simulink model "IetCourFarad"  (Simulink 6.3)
settings: Solver=ode45  StartTime=0.0  StopTime=5E-4  RelTol=1e-3
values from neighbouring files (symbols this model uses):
  beta = 0.95    [Constantes.m]    (also in ConstantesBck.m; ResCourV1.m = 1; ResCrV1.m = 1; ResEnerV1.m = 1)
undefined symbols (not defined in the file or in its folder): ln
libraries: simulink x1

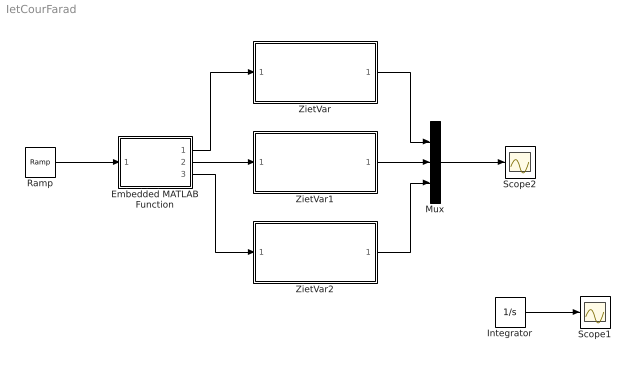
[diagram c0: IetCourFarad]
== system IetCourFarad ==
  Embedded MATLAB Function : Stateflow chart
  Integrator : Integrator
  Mux : Mux  Inputs=3
  Ramp : simulink/Sources/Ramp  slope=1  start=0  X0=0
  Scope1 : Scope
  Scope2 : Scope
  ZietVar : Subsystem
  ZietVar1 : Subsystem
  ZietVar2 : Subsystem
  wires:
  Ramp/1 -> Embedded MATLAB Function/1(u)
  Embedded MATLAB Function/1(Icar) -> ZietVar/1(Istim)
  ZietVar/1(If) -> Mux/1
  Integrator/1 -> Scope1/1
  Embedded MATLAB Function/2(Isin) -> ZietVar1/1(Istim)
  Embedded MATLAB Function/3(Isint) -> ZietVar2/1(Istim)
  ZietVar1/1(If) -> Mux/2
  ZietVar2/1(If) -> Mux/3
  Mux/1 -> Scope2/1

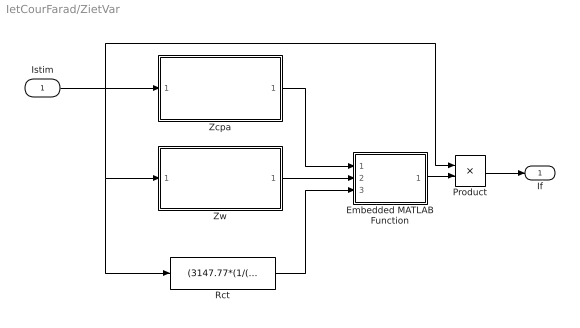
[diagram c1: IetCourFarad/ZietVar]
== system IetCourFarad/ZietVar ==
  Istim : Inport
  Embedded MATLAB Function : Stateflow chart
  Product : Product
  Rct : Fcn  Expr=(3147.77*(1/((1E6*abs(u))^0.7199)))*1000
  Zcpa : Subsystem
  Zw : Subsystem
  If : Outport
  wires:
  Istim/1 -> Zw/1(InZw), Rct/1, Zcpa/1(InZcpa), Product/1
  Product/1 -> If/1
  Embedded MATLAB Function/1(Zdiv) -> Product/2
  Zcpa/1(OutZcpa) -> Embedded MATLAB Function/1(Zcpa)
  Zw/1(OutZw) -> Embedded MATLAB Function/2(Zw)
  Rct/1 -> Embedded MATLAB Function/3(Rct)

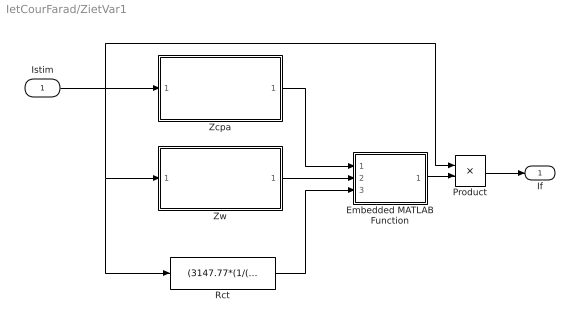
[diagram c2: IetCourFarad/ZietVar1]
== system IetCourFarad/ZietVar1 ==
  Istim : Inport
  Embedded MATLAB Function : Stateflow chart
  Product : Product
  Rct : Fcn  Expr=(3147.77*(1/((1E6*abs(u))^0.7199)))*1000
  Zcpa : Subsystem
  Zw : Subsystem
  If : Outport
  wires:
  Istim/1 -> Zw/1(InZw), Rct/1, Zcpa/1(InZcpa), Product/1
  Product/1 -> If/1
  Embedded MATLAB Function/1(Zdiv) -> Product/2
  Zcpa/1(OutZcpa) -> Embedded MATLAB Function/1(Zcpa)
  Zw/1(OutZw) -> Embedded MATLAB Function/2(Zw)
  Rct/1 -> Embedded MATLAB Function/3(Rct)

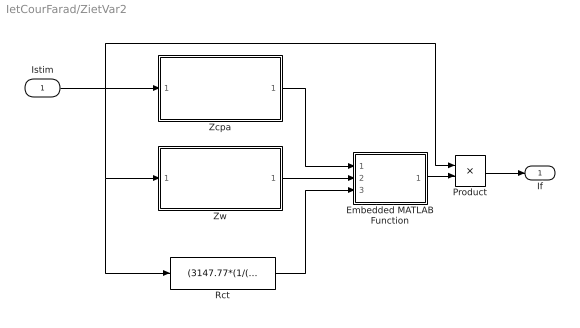
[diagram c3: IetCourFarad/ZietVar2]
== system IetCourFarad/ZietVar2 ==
  Istim : Inport
  Embedded MATLAB Function : Stateflow chart
  Product : Product
  Rct : Fcn  Expr=(3147.77*(1/((1E6*abs(u))^0.7199)))*1000
  Zcpa : Subsystem
  Zw : Subsystem
  If : Outport
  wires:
  Istim/1 -> Zw/1(InZw), Rct/1, Zcpa/1(InZcpa), Product/1
  Product/1 -> If/1
  Embedded MATLAB Function/1(Zdiv) -> Product/2
  Zcpa/1(OutZcpa) -> Embedded MATLAB Function/1(Zcpa)
  Zw/1(OutZw) -> Embedded MATLAB Function/2(Zw)
  Rct/1 -> Embedded MATLAB Function/3(Rct)

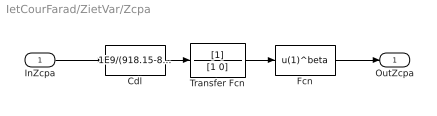
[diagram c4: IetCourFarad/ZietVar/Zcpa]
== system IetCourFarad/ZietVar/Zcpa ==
  InZcpa : Inport
  Cdl : Fcn  Expr=1E9/(918.15-80.854*ln(abs(u)*1E6))
  Fcn : Fcn  Expr=u(1)^beta
  Transfer Fcn : TransferFcn  Denominator=[1 0]
  OutZcpa : Outport
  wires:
  Transfer Fcn/1 -> Fcn/1
  Fcn/1 -> OutZcpa/1
  Cdl/1 -> Transfer Fcn/1
  InZcpa/1 -> Cdl/1

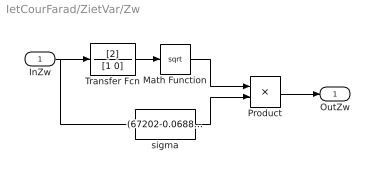
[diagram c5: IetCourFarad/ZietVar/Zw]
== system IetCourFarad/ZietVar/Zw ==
  InZw : Inport
  Math Function : Math  Operator=sqrt
  Product : Product
  Transfer Fcn : TransferFcn  Numerator=[2]  Denominator=[1 0]
  sigma : Fcn  Expr=(67202-0.0688*((1E6*abs(u))^2)-11.273*(1E6*abs(u)))
  OutZw : Outport
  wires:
  Transfer Fcn/1 -> Math Function/1
  InZw/1 -> Transfer Fcn/1, sigma/1
  Math Function/1 -> Product/1
  sigma/1 -> Product/2
  Product/1 -> OutZw/1

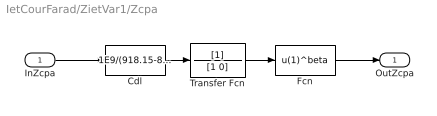
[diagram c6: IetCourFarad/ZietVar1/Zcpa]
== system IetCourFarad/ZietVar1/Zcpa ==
  InZcpa : Inport
  Cdl : Fcn  Expr=1E9/(918.15-80.854*ln(abs(u)*1E6))
  Fcn : Fcn  Expr=u(1)^beta
  Transfer Fcn : TransferFcn  Denominator=[1 0]
  OutZcpa : Outport
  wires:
  Transfer Fcn/1 -> Fcn/1
  Fcn/1 -> OutZcpa/1
  Cdl/1 -> Transfer Fcn/1
  InZcpa/1 -> Cdl/1

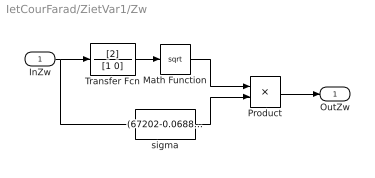
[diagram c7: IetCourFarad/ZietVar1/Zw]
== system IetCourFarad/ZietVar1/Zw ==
  InZw : Inport
  Math Function : Math  Operator=sqrt
  Product : Product
  Transfer Fcn : TransferFcn  Numerator=[2]  Denominator=[1 0]
  sigma : Fcn  Expr=(67202-0.0688*((1E6*abs(u))^2)-11.273*(1E6*abs(u)))
  OutZw : Outport
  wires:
  Transfer Fcn/1 -> Math Function/1
  InZw/1 -> Transfer Fcn/1, sigma/1
  Math Function/1 -> Product/1
  sigma/1 -> Product/2
  Product/1 -> OutZw/1

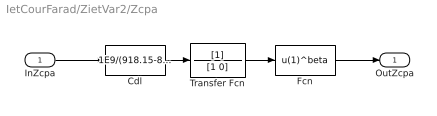
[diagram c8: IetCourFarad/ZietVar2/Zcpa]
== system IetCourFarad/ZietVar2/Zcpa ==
  InZcpa : Inport
  Cdl : Fcn  Expr=1E9/(918.15-80.854*ln(abs(u)*1E6))
  Fcn : Fcn  Expr=u(1)^beta
  Transfer Fcn : TransferFcn  Denominator=[1 0]
  OutZcpa : Outport
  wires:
  Transfer Fcn/1 -> Fcn/1
  Fcn/1 -> OutZcpa/1
  Cdl/1 -> Transfer Fcn/1
  InZcpa/1 -> Cdl/1

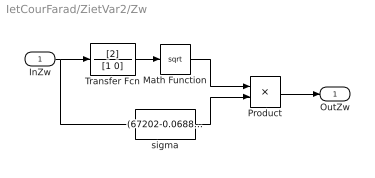
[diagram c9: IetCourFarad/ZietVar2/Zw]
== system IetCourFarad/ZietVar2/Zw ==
  InZw : Inport
  Math Function : Math  Operator=sqrt
  Product : Product
  Transfer Fcn : TransferFcn  Numerator=[2]  Denominator=[1 0]
  sigma : Fcn  Expr=(67202-0.0688*((1E6*abs(u))^2)-11.273*(1E6*abs(u)))
  OutZw : Outport
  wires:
  Transfer Fcn/1 -> Math Function/1
  InZw/1 -> Transfer Fcn/1, sigma/1
  Math Function/1 -> Product/1
  sigma/1 -> Product/2
  Product/1 -> OutZw/1

== matlab function ZietVar/Embedded
MATLAB Function ==
function Zdiv = fcn(Zcpa,Zw,Rct)
% This block supports an embeddable subset of the MATLAB language.
% See the help menu for details. 

Zf=1/(1/Zw+1/Rct);
Zdiv = 1/(1+Zf/Zcpa);

== matlab function Embedded
MATLAB Function ==
function [Icar,Isin,Isint] = fcn(u)
% This block supports an embeddable subset of the MATLAB language.
% See the help menu for details. 

T0 = 1E-4;

if u >= 0 && u < T0
    Icar = 1E-6;
    Isin = 1E-6*sin(pi/T0*u);
    Isint = 1E-6*sin(pi/(2*T0)*u);
else 
    Icar = 0;
    Isin = 0;
    Isint = 0;
end;

== matlab function ZietVar1/Embedded
MATLAB Function ==
function Zdiv = fcn(Zcpa,Zw,Rct)
% This block supports an embeddable subset of the MATLAB language.
% See the help menu for details. 

Zf=1/(1/Zw+1/Rct);
Zdiv = 1/(1+Zf/Zcpa);

== matlab function ZietVar2/Embedded
MATLAB Function ==
function Zdiv = fcn(Zcpa,Zw,Rct)
% This block supports an embeddable subset of the MATLAB language.
% See the help menu for details. 

Zf=1/(1/Zw+1/Rct);
Zdiv = 1/(1+Zf/Zcpa);
